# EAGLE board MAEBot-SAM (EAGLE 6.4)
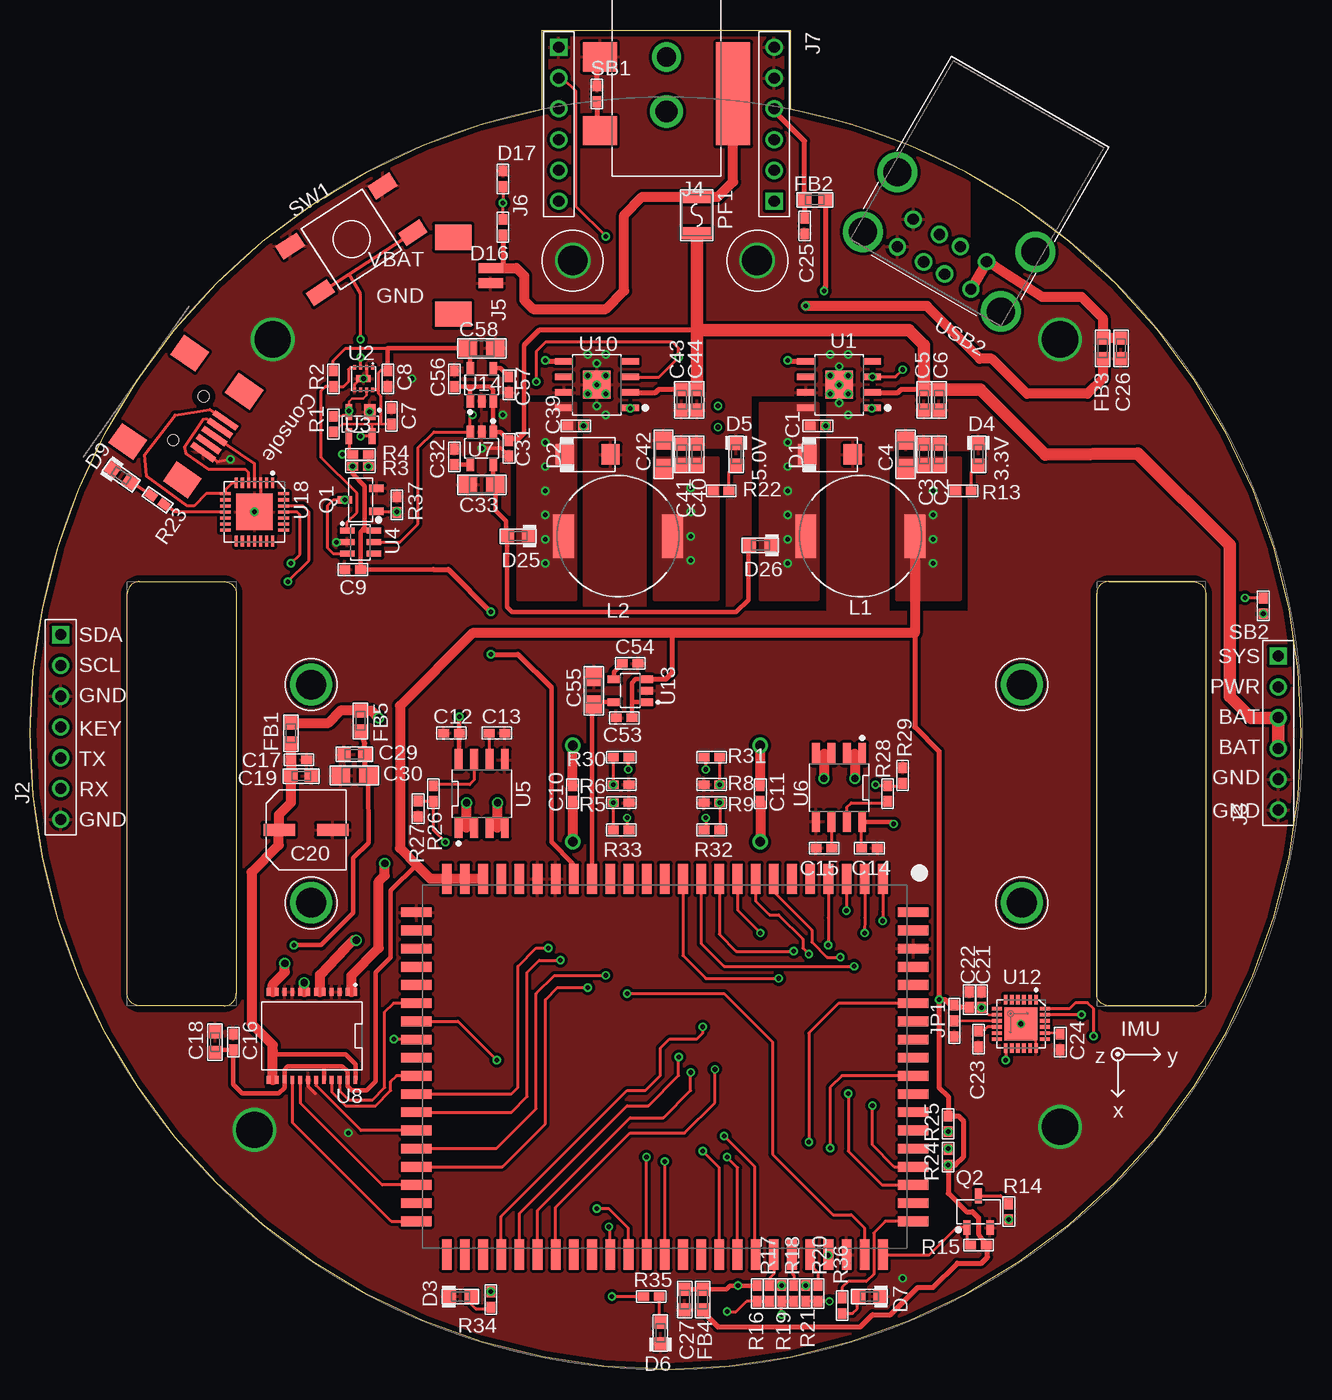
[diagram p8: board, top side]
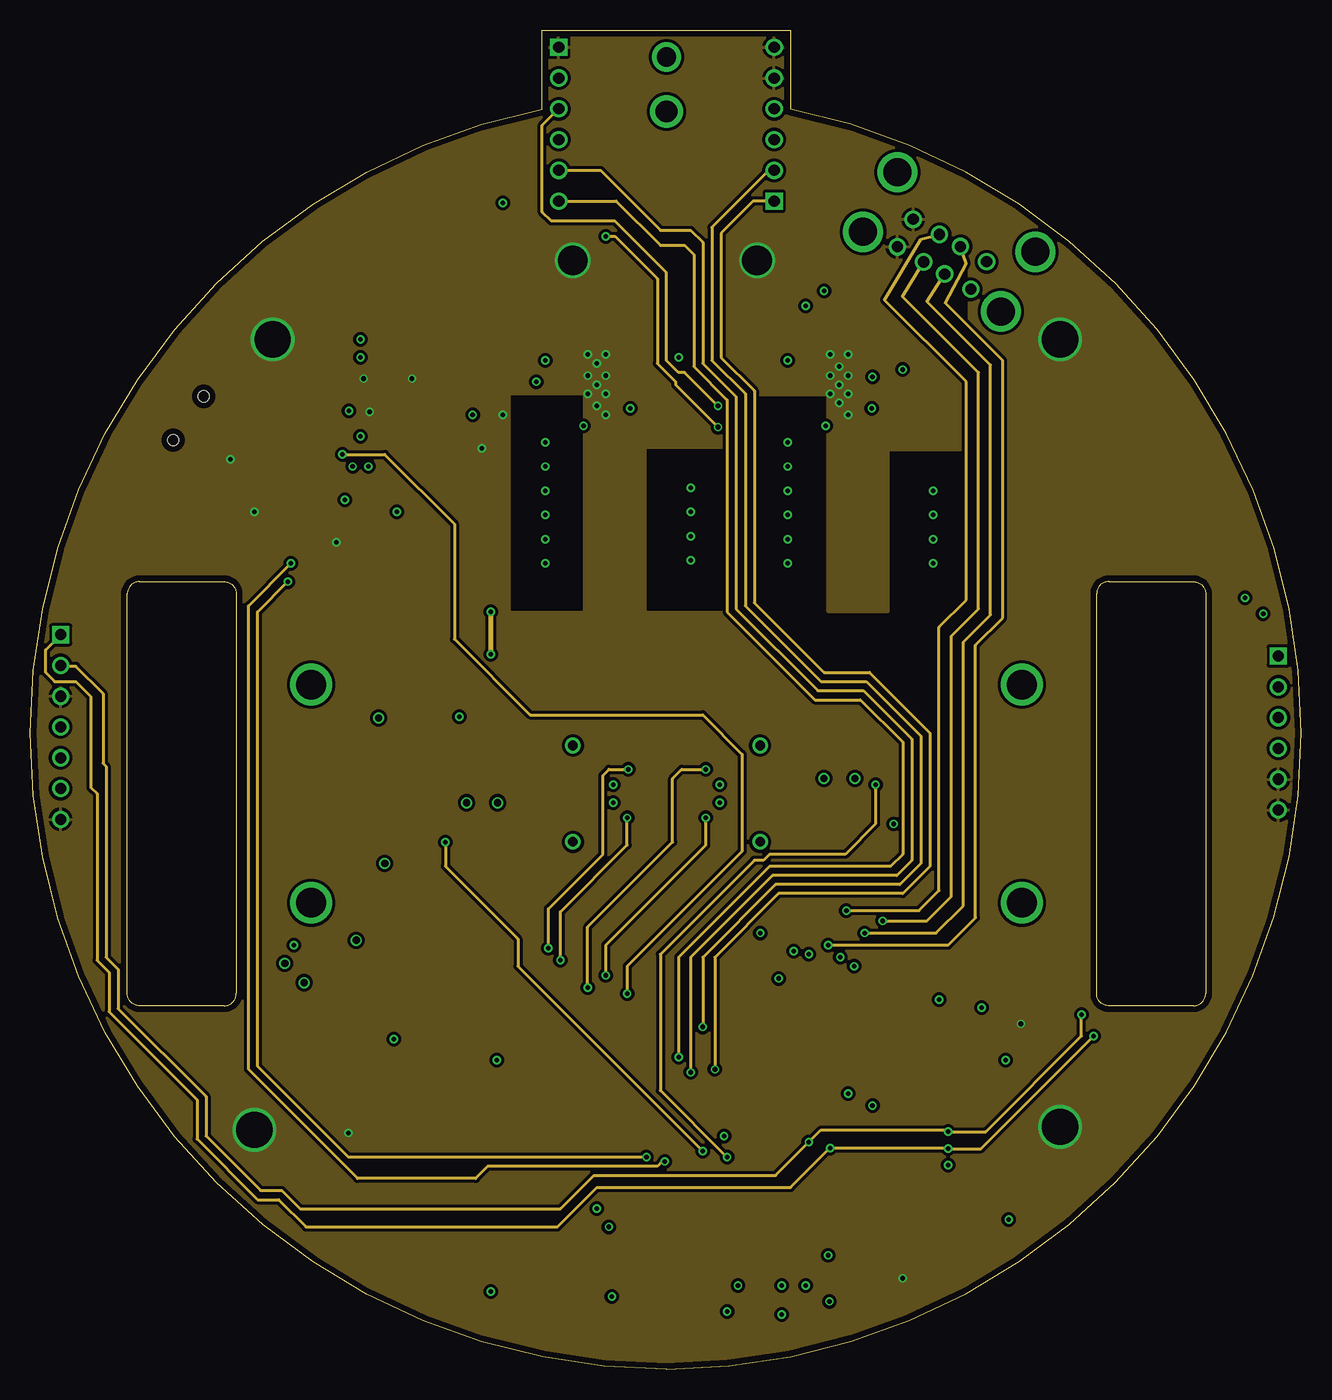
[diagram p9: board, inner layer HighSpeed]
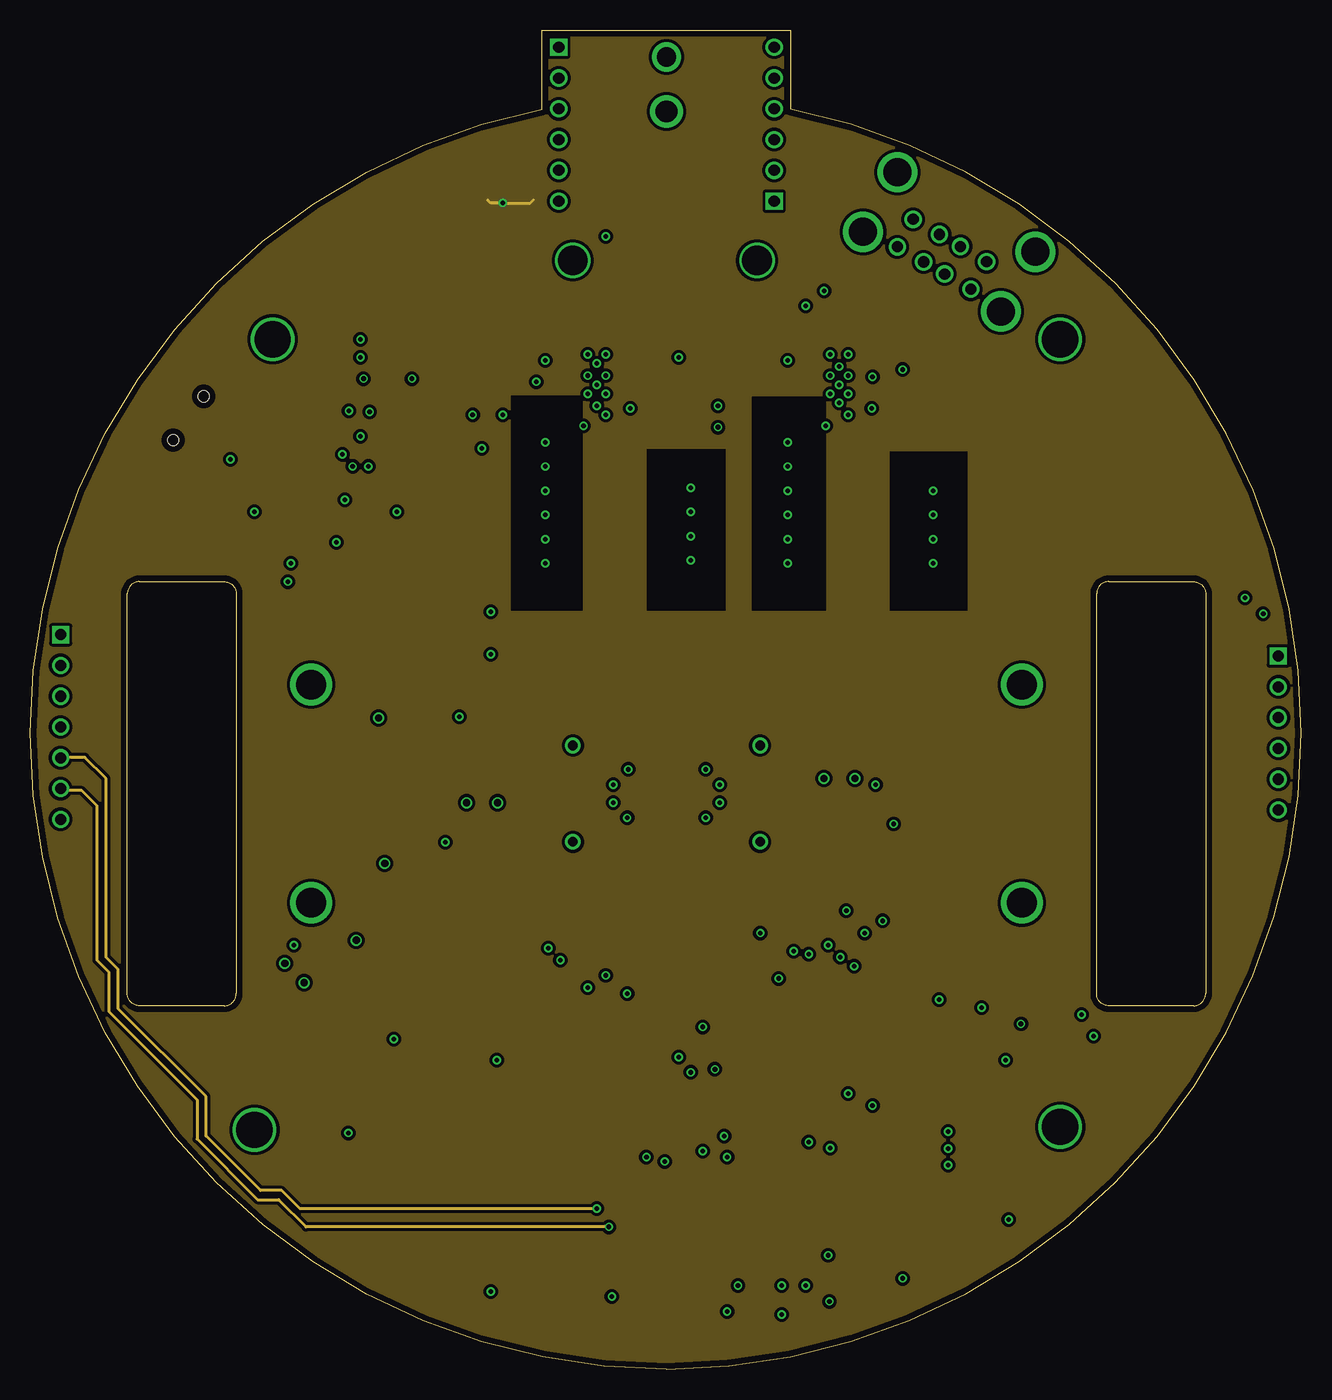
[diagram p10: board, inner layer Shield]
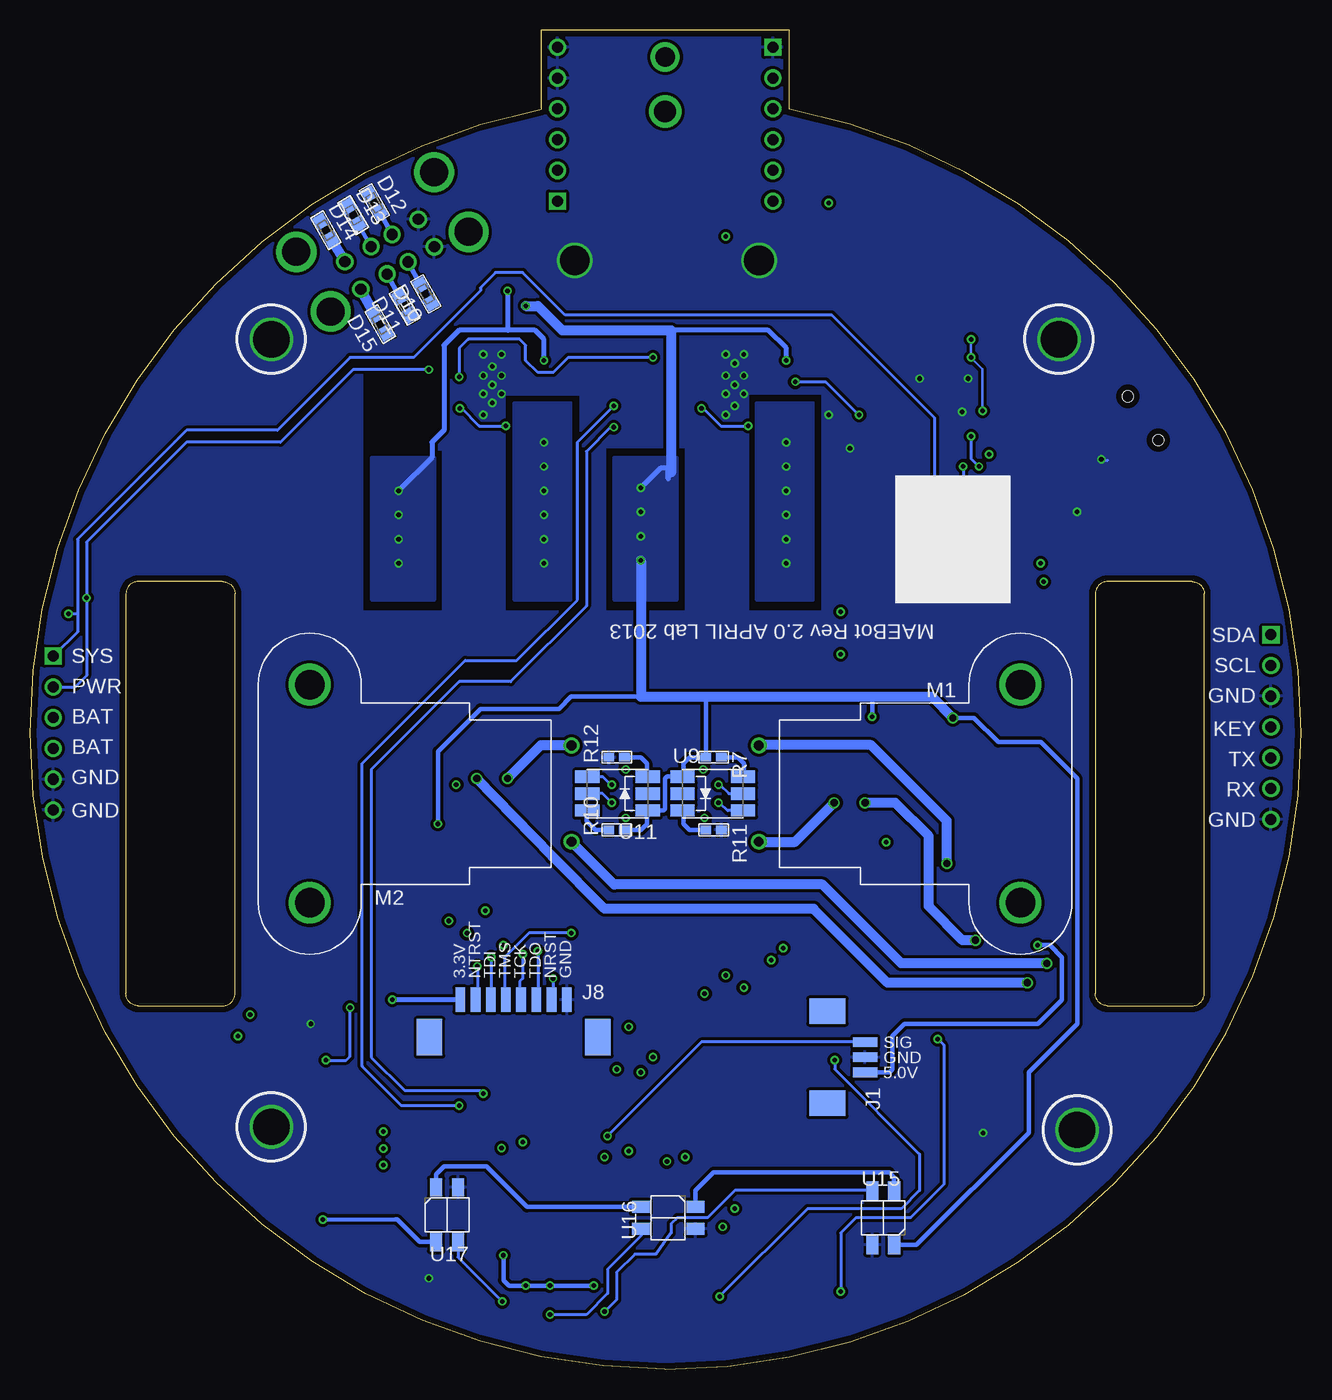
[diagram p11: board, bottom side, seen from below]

Size 104.9 x 110.5 mm. Coordinates in mm from the lower left corner, seen from the top.
Outline: 9.01,65 16.01,65 arc-90 17.01,64 17.01,31 arc-90 16.01,30 9.01,30 arc-90 8.01,31 8.01,64 arc-90 9.01,65
Outline: 89.01,65 96.01,65 arc-90 97.01,64 97.01,31 arc-90 96.01,30 89.01,30 arc-90 88.01,31 88.01,64 arc-90 89.01,65
Outline: 42.26,104 42.26,110.5 62.76,110.5 62.76,104 arc-168 52.51,0 arc-169 42.26,104
Copper layers (1*2+15*16): Top 0.035mm / dielectric 0.15mm / HighSpeed 0.035mm / dielectric 1.1mm / Shield 0.035mm / dielectric 0.15mm / Bottom 0.035mm
Design rules "default *": minimum track width 6mil, minimum drill 15mil, track to track 6mil, track to pad 6mil, pad to pad 6mil, via to via 6mil, smd to smd 0mil, copper to edge 20mil, drill to drill 8mil, minimum pad ring 10mil, minimum via ring 6mil, stop-mask expansion 0mil, vias tented up to drill 16mil, thermal gap 10mil

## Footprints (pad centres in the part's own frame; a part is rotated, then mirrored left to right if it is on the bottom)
R0402 = smd 0.711 x 0.889: P$1 0,0.648; P$2 0,-0.648
SM0603 = smd 1.1 x 1: P$1 -0.85,0; P$2 0.85,0
SM0805 = smd 1.4 x 1.52: P$1 0,1.14; P$2 0,-1.14
VS_SERIES_D8 = smd 2.6 x 1: N 2.2,0; P -2.2,0
SSA33L = smd 1.52 x 1.68: AN -1.88,0; CATH 1.88,0
D0603 = smd 1 x 1.09: AN 0,-0.89; CATH 0,0.89
PICO-3 = smd 2.1 x 3: M$1 -3.8,-3.1; M$2 3.8,-3.1 | smd 0.8 x 2: P$1 -1.25,0; P$2 0,0; P$3 1.25,0
J7X1 = drill 0.914 square: P$1 0,7.62 | drill 0.914: P$2 0,5.08; P$3 0,2.54; P$4 0,0; P$5 0,-2.54; P$6 0,-5.08; P$7 0,-7.62
J6X1 = drill 0.914 square: P$1 0,6.35 | drill 0.914: P$2 0,3.81; P$3 0,1.27; P$4 0,-1.27; P$5 0,-3.81; P$6 0,-6.35
PJ-002A-SMT = drill 1.6: M$1 0,-3.05 | drill 1.8: M$2 0,1.45 | smd 2.8 x 8.5: P$1 -5.5,0 | smd 2.8 x 2.4: P$2 5.5,-3.05; P$3 5.5,3.05
PICO-2 = smd 2.1 x 3: M$1 -3.175,-3.1; M$2 3.175,-3.1 | smd 0.8 x 2: P$1 -0.625,0; P$2 0.625,0
PICO-8 = smd 2.1 x 3: M$1 -6.945,-3.1; M$2 6.945,-3.1 | smd 0.8 x 2: P$1 -4.395,0; P$2 -3.145,0; P$3 -1.895,0; P$4 -0.645,0; P$5 0.605,0; P$6 1.855,0; P$7 3.125,0; P$8 4.395,0
JP0402 = smd 0.711 x 0.889: IN 0,0; OUT1 0,1.296; OUT2 0,-1.296
VLF10040_SERIES = smd 1.7 x 3.6: P$1 -4.5,0; P$2 4.5,0
MMG_MOTOR = drill 0.8: P$1 -3.97,0; P$2 3.97,0 | drill 2.44: P$3 9,-21.6; P$4 -9,-21.6
1210L_SERIES = smd 1 x 2.5: P$1 -1.5,0; P$2 1.5,0
SOT23 = smd 0.6 x 1.2: P$1 -0.95,-1.31; P$2 0.95,-1.31; P$3 0,1.31
SAMA5_CARRIER = smd 0.8 x 2.5: P$1 2,-0.5; P$2 3.5,-0.5; P$3 5,-0.5; P$4 6.5,-0.5; P$5 8,-0.5; P$6 9.5,-0.5; P$7 11,-0.5; P$8 12.5,-0.5; P$9 14,-0.5; P$10 15.5,-0.5; P$11 17,-0.5; P$12 18.5,-0.5; P$13 20,-0.5; P$14 21.5,-0.5; P$15 23,-0.5; P$16 24.5,-0.5; P$17 26,-0.5; P$18 27.5,-0.5; P$19 29,-0.5; P$20 30.5,-0.5; P$21 32,-0.5; P$22 33.5,-0.5; P$23 35,-0.5; P$24 36.5,-0.5; P$25 38,-0.5; P$44 38,30.5; P$45 36.5,30.5; P$46 35,30.5; P$47 33.5,30.5; P$48 32,30.5; P$49 30.5,30.5; P$50 29,30.5; P$51 27.5,30.5; P$52 26,30.5; P$53 24.5,30.5; P$54 23,30.5; P$55 21.5,30.5; P$56 20,30.5; P$57 18.5,30.5; P$58 17,30.5; P$59 15.5,30.5; P$60 14,30.5; P$61 12.5,30.5; P$62 11,30.5; P$63 9.5,30.5; P$64 8,30.5; P$65 6.5,30.5; P$66 5,30.5; P$67 3.5,30.5; P$68 2,30.5 | smd 2.5 x 0.8: P$26 40.5,2.25; P$27 40.5,3.75; P$28 40.5,5.25; P$29 40.5,6.75; P$30 40.5,8.25; P$31 40.5,9.75; P$32 40.5,11.25; P$33 40.5,12.75; P$34 40.5,14.25; P$35 40.5,15.75; P$36 40.5,17.25; P$37 40.5,18.75; P$38 40.5,20.25; P$39 40.5,24.75; P$40 40.5,23.25; P$41 40.5,21.75; P$42 40.5,26.25; P$43 40.5,27.75; P$69 -0.5,27.75; P$70 -0.5,26.25; P$71 -0.5,24.75; P$72 -0.5,23.25; P$73 -0.5,21.75; P$74 -0.5,20.25; P$75 -0.5,18.75; P$76 -0.5,17.25; P$77 -0.5,15.75; P$78 -0.5,14.25; P$79 -0.5,12.75; P$80 -0.5,11.25; P$81 -0.5,9.75; P$82 -0.5,8.25; P$83 -0.5,6.75; P$84 -0.5,5.25; P$85 -0.5,3.75; P$86 -0.5,2.25
FSMJSMA = smd 1.3 x 2.1: P$1 -2.3,4.55; P$2 -2.3,-4.55; P$3 2.3,4.55; P$4 2.3,-4.55
RD-8-1 = smd 0.55 x 1.49: P$1 -1.92,-2.72; P$2 -0.64,-2.72; P$3 0.64,-2.72; P$4 1.92,-2.72; P$5 1.92,2.72; P$6 0.64,2.72; P$7 -0.64,2.72; P$8 -1.92,2.72 | smd 2.29 x 2.29: P$9 0,0
MLF8 = smd 0.35 x 0.25: P$1 -0.925,0.75; P$2 -0.925,0.25; P$3 -0.925,-0.25; P$4 -0.925,-0.75; P$5 0.925,-0.75; P$6 0.925,-0.25; P$7 0.925,0.25; P$8 0.925,0.75 | smd 0.6 x 1.2: P$9 0,0
90-0183 = smd 0.94 x 1.31: P$1 -0.765,-1 | smd 0.55 x 1.31: P$2 0.96,-1; P$3 0.96,1; P$4 -0.96,1
90-0240 = smd 1.2 x 0.5: P$1 -1.1,0.95; P$2 -1.1,0; P$3 -1.1,-0.95; P$4 1.1,-0.95; P$5 1.1,0; P$6 1.1,0.95
LC_8-PIN_SOIC = smd 0.65 x 1.75: P$1 -1.905,-2.8; P$2 -0.635,-2.8; P$3 0.635,-2.8; P$4 1.905,-2.8; P$5 1.905,2.8; P$6 0.635,2.8; P$7 -0.635,2.8; P$8 -1.905,2.8
R-PDS0-G5_(SOT23-5) = smd 0.6 x 1.05: P$1 -0.95,-1.35; P$2 0,-1.35; P$3 0.95,-1.35; P$4 0.95,1.35; P$5 -0.95,1.35
SSOP24-P-300-0.65A = smd 0.32 x 0.65: P$1 -3.575,-3.625; P$2 -2.925,-3.625; P$3 -2.275,-3.625; P$4 -1.625,-3.625; P$5 -0.975,-3.625; P$6 -0.325,-3.625; P$7 0.325,-3.625; P$8 0.975,-3.625; P$9 1.625,-3.625; P$10 2.275,-3.625; P$11 2.925,-3.625; P$12 3.575,-3.625; P$13 3.575,3.625; P$14 2.925,3.625; P$15 2.275,3.575; P$16 1.625,3.625; P$17 0.975,3.625; P$18 0.325,3.625; P$19 -0.325,3.625; P$20 -0.975,3.625; P$21 -1.625,3.625; P$22 -2.275,3.625; P$23 -2.925,3.625; P$24 -3.575,3.625
EE-SX1131 = smd 2 x 1: AN -2.5,1.4; C 2.5,1.4; CA -2.5,-1.4; E1 2.5,0; E2 2.5,-1.4; NC -2.5,0
MPU-60X0 = smd 0.8 x 0.3: P$1 -2,1.25; P$2 -2,0.75; P$3 -2,0.25; P$4 -2,-0.25; P$5 -2,-0.75; P$6 -2,-1.25; P$13 2,-1.25; P$14 2,-0.75; P$15 2,-0.25; P$16 2,0.25; P$17 2,0.75; P$18 2,1.25 | smd 0.3 x 0.8: P$7 -1.25,-1.975; P$8 -0.75,-1.975; P$9 -0.25,-1.975; P$10 0.25,-1.975; P$11 0.75,-1.975; P$12 1.25,-1.975; P$19 1.25,1.975; P$20 0.75,1.975; P$21 0.25,1.975; P$22 -0.25,1.975; P$23 -0.75,1.975; P$24 -1.25,1.975 | smd 2.7 x 2.7: P$25 0,0
ADP171X_(SOT23-5) = smd 0.6 x 1.05: P$1 -0.95,-1.35; P$2 0,-1.35; P$3 0.95,-1.35; P$4 0.95,1.35; P$5 -0.95,1.35
QRE1113GR = smd 1 x 1.5: P$1 0.9,-2.25; P$2 0.9,2.25; P$3 -0.9,2.25; P$4 -0.9,-2.25
28QFN-5MM = smd 0.9 x 0.25: P$1 -2.4,1.5; P$2 -2.4,1; P$3 -2.4,0.5; P$4 -2.4,0; P$5 -2.4,-0.5; P$6 -2.4,-1; P$7 -2.4,-1.5; P$15 2.4,-1.5; P$16 2.4,-1; P$17 2.4,-0.5; P$18 2.4,0; P$19 2.4,0.5; P$20 2.4,1; P$21 2.4,1.5 | smd 0.25 x 0.9: P$8 -1.5,-2.4; P$9 -1,-2.4; P$10 -0.5,-2.4; P$11 0,-2.4; P$12 0.5,-2.4; P$13 1,-2.4; P$14 1.5,-2.4; P$22 1.5,2.4; P$23 1,2.4; P$24 0.5,2.4; P$25 0,2.4; P$26 -0.5,2.4; P$27 -1,2.4; P$28 -1.5,2.4 | smd 3 x 3: P$29 0,0
USB_MINI_A = smd 2.3 x 0.5: D_N 7.85,0.8; D_P 7.85,0; GND 7.85,-1.6; ID 7.85,-0.8; VBUS 7.85,1.6 | smd 2.5 x 2: M1 2.25,4.45; M2 7.75,4.45; M3 7.75,-4.45; M4 2.25,-4.45 | hole 0.9: 5.25,2.2; 5.25,-2.2
XM7A-0442-A = drill 0.92: BOT_D_N -1,2.71; BOT_D_P 1,2.71; BOT_GND 3.5,2.71; BOT_VBUS -3.5,2.71; TOP_D_N -1,5.33; TOP_D_P 1,5.33; TOP_GND 3.5,5.33; TOP_VBUS -3.5,5.33 | drill 2.3: M1 -6.57,0; M2 -6.57,5.68; M3 6.57,5.68; M4 6.57,0

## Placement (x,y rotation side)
C1  0.1uF  [R0402]  65.01,77.85 270 top
C2  22uF  [SM0603]  75.01,75.5 270 top
C3  22uF  [SM0603]  73.76,75.5 270 top
C4  47uF  [SM0805]  72.26,75.5 0 top
C5  10uF  [SM0603]  73.76,80 90 top
C6  10uF  [SM0603]  75.01,80 90 top
C7  0.1uF  [R0402]  29.81,78.65 0 top
C8  0.1uF  [R0402]  29.51,81.75 0 top
C9  0.1uF  [R0402]  26.61,66 90 top
C10  0.1uF  [R0402]  44.76,47.5 0 top
C11  0.1uF  [R0402]  60.26,47.5 0 top
C12  0.1uF  [R0402]  34.76,52.5 90 top
C13  1000pF  [R0402]  38.51,52.5 270 top
C14  0.1uF  [R0402]  69.26,43 270 top
C15  1000pF  [R0402]  65.51,43 90 top
C16  0.1uF  [R0402]  16.76,27 0 top
C17  0.1uF  [R0402]  22.16,50.3 270 top
C18  10uF  [SM0603]  15.26,27 270 top
C19  10uF  [SM0603]  22.36,48.95 180 top
C20  220uF  [VS_SERIES_D8]  22.76,44.5 0 top
C21  0.1uF  [R0402]  78.51,30.5 0 top
C22  0.01uF  [R0402]  77.51,30.5 0 top
C23  0.1uF  [R0402]  78.26,27.25 180 top
C24  2200pF  [R0402]  85.01,27 180 top
C25  0.1uF  [R0402]  63.91,94.35 180 top
C26  22uF  [SM0603]  90.01,84.25 90 top
C27  22uF  [SM0603]  54.01,5.75 90 top
C29  10uF  [SM0603]  26.76,50.75 0 top
C30  47uF  [SM0805]  26.76,49 90 top
C31  1uF  [R0402]  39.51,76 180 top
C32  0.01uF  [R0402]  35.01,75.3 0 top
C33  10uF  [SM0805]  37.26,73 90 top
C39  0.1uF  [R0402]  45.01,77.85 270 top
C40  22uF  [SM0603]  55.01,75.5 270 top
C41  22uF  [SM0603]  53.76,75.5 270 top
C42  47uF  [SM0805]  52.26,75.5 0 top
C43  10uF  [SM0603]  53.76,80 90 top
C44  10uF  [SM0603]  55.01,80 90 top
C53  2.2uF, 6.3V, X5R  [R0402]  49.01,53.75 90 top
C54  0.01uF  [R0402]  49.51,58.25 270 top
C55  2.2uF, 6.3V, X5R  [SM0805]  46.51,56 0 top
C56  1uF  [R0402]  35.01,81.75 0 top
C57  0.01uF  [R0402]  39.51,81.25 180 top
C58  10uF  [SM0805]  37.26,84.25 270 top
D1  SSA33L  [SSA33L]  66.01,75.5 180 top
D2  SSA33L  [SSA33L]  46.01,75.5 180 top
D3  GRN  [D0603]  35.51,6 90 top
D4  GRN  [D0603]  78.26,75.5 0 top
D5  GRN  [D0603]  58.26,75.5 0 top
D6  GRN  [D0603]  52.01,3 180 top
D7  GRN  [D0603]  69.26,6 270 top
D9  BLUE  [D0603]  7.51,73.75 55 top
D10  PGB1010603MR  [SM0603]  72.26,88.75 120 bottom
D11  PGB1010603MR  [SM0603]  74.01,87.75 120 bottom
D12  PGB1010603MR  [SM0603]  76.51,96.25 300 bottom
D13  PGB1010603MR  [SM0603]  78.26,95.25 300 bottom
D14  PGB1010603MR  [SM0603]  80.51,94 300 bottom
D15  PGB1010603MR  [SM0603]  76.01,86.25 120 bottom
D16  PGB1010402KR  [R0402]  39.01,94.25 180 top
D17  PGB1010402KR  [R0402]  39.01,98.25 0 top
D25  [D0603]  40.26,68.75 270 top
D26  [D0603]  60.26,68 270 top
FB1  200R 2.2A  [SM0603]  21.51,52.5 90 top
FB2  200R 2.2A  [SM0603]  64.76,96.5 180 top
FB3  200R 2.2A  [SM0603]  88.51,84.25 90 top
FB4  200R 2.2A  [SM0603]  55.51,5.75 90 top
FB5  200R 2.2A  [SM0603]  27.26,53.5 270 top
J1  IR Range Finder  [PICO-3]  36.01,25.75 270 bottom
J2  To Variscite  [J7X1]  2.51,53 0 top
J3  POWER  [J6X1]  103.01,52.5 0 top
J4  PJ-002A-SMT  [PJ-002A-SMT]  52.51,105.25 180 top
J5  Battery IN  [PICO-2]  38.01,90.25 270 top
J6  Radio-A  [J6X1]  43.62,102.75 0 top
J7  Radio-B  [J6X1]  61.4,102.75 180 top
J8  JTAG  [PICO-8]  65.01,30.5 0 bottom
JP1  JP0402  [JP0402]  76.26,28.75 180 top
L1  3.3uH  [VLF10040_SERIES]  68.51,68.75 0 top
L2  3.3uH  [VLF10040_SERIES]  48.51,68.75 0 top
M1  50:1  [MMG_MOTOR]  44.78,47.5 270 top
M2  50:1  [MMG_MOTOR]  60.24,47.5 90 top
PF1  1210L200 - 4A  [1210L_SERIES]  55.01,95.25 270 top
Q1  2N7002  [SOT23]  27.26,71.75 90 top
Q2  2N7002  [SOT23]  78.26,13 0 top
R1  20K  [R0402]  25.01,78 0 top
R2  10K  [R0402]  25.01,81.75 180 top
R3  100K  [R0402]  27.26,74.5 270 top
R4  10K  [R0402]  27.26,75.5 270 top
R5  6.8K  [R0402]  48.76,46.75 270 top
R6  6.8K  [R0402]  48.76,48.25 270 top
R7  0  [R0402]  48.51,50.5 270 bottom
R8  6.8K  [R0402]  56.26,48.25 90 top
R9  6.8K  [R0402]  56.26,46.75 90 top
R10  0  [R0402]  56.51,44.5 90 bottom
R11  384  [R0402]  48.51,44.5 270 bottom
R12  384  [R0402]  56.51,50.5 90 bottom
R13  56  [R0402]  77.01,72.5 270 top
R14  220  [R0402]  80.76,13 0 top
R15  100K  [R0402]  78.26,10.25 90 top
R16  47K  [R0402]  60.01,6.25 180 top
R17  0  [R0402]  61.01,6.25 180 top
R18  0  [R0402]  63.01,6.25 180 top
R19  47K  [R0402]  62.01,6.25 180 top
R20  0  [R0402]  65.01,6.25 180 top
R21  47K  [R0402]  64.01,6.25 180 top
R22  56  [R0402]  57.01,72.5 270 top
R23  82  [R0402]  10.51,71.75 235 top
R24  4.7K  [R0402]  75.76,17.5 0 top
R25  4.7K  [R0402]  75.76,20.25 180 top
R26  TBD  [R0402]  33.26,47.5 0 top
R27  TBD  [R0402]  32.01,46.25 180 top
R28  TBD  [R0402]  70.76,47.5 0 top
R29  TBD  [R0402]  72.01,49 180 top
R30  0  [R0402]  48.76,50.5 90 top
R31  0  [R0402]  56.26,50.5 270 top
R32  0  [R0402]  56.26,44.5 270 top
R33  0  [R0402]  48.76,44.5 90 top
R34  56  [R0402]  38.01,5.75 180 top
R35  56  [R0402]  51.26,6 270 top
R36  56  [R0402]  67.01,5.25 180 top
R37  100K  [R0402]  30.26,71.35 0 top
SAMA1  SAMA5_CARRIER  [SAMA5_CARRIER]  72.37,39.96 180 top
SB1  SB0402  [R0402]  46.76,105.25 0 top
SB2  SB0402  [R0402]  101.76,63 180 top
SW1  FSMSMTR  [FSMJSMA]  26.51,93.25 303 top
U1  ADP2303ADRZ-3.3-R7  [RD-8-1]  66.76,81.25 90 top
U2  MIC2788  [MLF8]  27.51,81.75 270 top
U3  MAX6816  [90-0183]  27.26,78 180 top
U4  MAX16045  [90-0240]  27.26,68.25 0 top
U5  ACS714 +/- 5A  [LC_8-PIN_SOIC]  37.26,47.5 0 top
U6  ACS714 +/- 5A  [LC_8-PIN_SOIC]  66.76,48 180 top
U7  LP2985-50DBVR  [R-PDS0-G5_(SOT23-5)]  37.26,76 180 top
U8  TB6612FNG  [SSOP24-P-300-0.65A]  23.26,27.5 180 top
U9  EE-SX1131  [EE-SX1131]  48.58,47.5 0 bottom
U10  ADP2303ADRZ-5.0-R7  [RD-8-1]  46.76,81.25 90 top
U11  EE-SX1131  [EE-SX1131]  56.44,47.5 180 bottom
U12  MPU-6050  [MPU-60X0]  81.76,28.5 270 top
U13  ADP1713AUJZ-2.5-R7  [ADP171X_(SOT23-5)]  49.51,56 90 top
U14  LP2985-33DBVR  [R-PDS0-G5_(SOT23-5)]  37.26,81.25 0 top
U15  QRE1113GR  [QRE1113GR]  34.51,12.5 0 bottom
U16  QRE1113GR  [QRE1113GR]  52.26,12.5 90 bottom
U17  QRE1113GR  [QRE1113GR]  70.51,12.75 180 bottom
U18  CP2102  [28QFN-5MM]  18.51,70.75 270 top
USB1  USB_MINI_A  [USB_MINI_A]  8.76,81.5 325 top
USB2  XM7A-0442-A  [XM7A-0442-A]  77.26,95.5 150 top

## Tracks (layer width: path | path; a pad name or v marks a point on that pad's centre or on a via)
3.3V  (via drill 0.38)
  Top 0.203: U12.P$8 79.11,29.25 C21.P$2
  Top 0.254: C22.P$2 C21.P$2 | U12.P$13 v80.51,25.5
  Top 0.381: C53.P$2 49.65,54.75 | 49.65,54.75 49.65,56.65 49.96,56.95 U13.P$3 | U13.P$1 49.7,55.05 49.65,54.75 | 24.26,25 25.76,25 26.18,24.57 U8.P$23 26.18,23.32 26.51,23 27.76,23 28.51,23.75 28.51,32.75 29.76,34 29.76,39.5 31.88,41.62 | 24.26,25 21.26,25 20.98,24.73 U8.P$15 20.98,23.23 20.51,22.75 17.51,22.75 16.76,23.5 C16.P$2 15.46,26.35 C18.P$2 | U8.P$20 24.23,24.98 24.26,25
  Top 0.406: U1.P$5 62.59,83.17 v62.51,83.25 | FB2.P$1 65.61,89.35 v65.51,89 | R24.P$2 76.36,16.85 77.01,17.5 77.01,20.5 76.61,20.9 R25.P$2 75.76,22.5 75.01,23.25 v75.01,30.5 | U13.P$3 52.46,56.95 53.01,57.5 53.01,60.75 | 73.01,60.75 73.01,53 75.01,51 v75.01,30.5 | C22.P$2 76.45,29.85 JP1.OUT2 75.96,30.05 75.51,30.5 v75.01,30.5 | R24.P$2 75.76,14.5 77.26,13 77.76,13 78.26,12.5 78.26,11.15 R15.P$2 79.01,10.15 79.01,9.25 78.51,8.75 76.51,8.75 74.51,6.75 73.26,6.75 71.01,4.5 69.51,4.5 68.51,3.5 56.76,3.5 55.51,4.75 FB4.P$1 | R24.P$2
  Top 0.813: SAMA1.P$23 SAMA1.P$24 SAMA1.P$25 34.33,40.5 33.01,40.5 31.88,41.62 30.51,43 30.51,54.75 36.51,60.75 53.01,60.75 73.01,60.75 L1.P$2
  Bottom 0.254: v80.51,25.5 78.82,25.5 78.51,25.82 C21.P$2
  Bottom 0.406: v62.51,83.25 62.51,85 63.26,85.75 65.51,85.75 | 65.51,85.75 69.51,85.75 70.76,84.5 70.76,77.5 71.76,76.5 71.76,75.25 v74.51,72.5 | v65.51,89 65.51,85.75 | J8.P$1 v75.01,30.5
  other vias: 74.51,70.5 74.51,68.5 74.51,66.5 78.51,29.85 75.76,16.85
  pour Top (no thermals): 71.51,75.25 76.76,75.25 76.76,63.5 71.51,63.5
  pour Bottom (no thermals): 71.51,75.25 76.76,75.25 76.76,63.5 71.51,63.5
3.3V_BYP
  Top 0.381: U14.P$4 38.8,82.6 C57.P$2
5.0V  (via drill 0.38, 0.6)
  Top 0.254: C14.P$2 68.61,45.15 U6.P$8
  Top 0.381: v35.41,53.85 v35.4,53.85 C12.P$2 35.4,50.35 U5.P$8 | 68.61,45.15 71.11,45.15 v71.26,45
  Top 0.406: U10.P$5 42.59,83.17 v42.51,83.25
  Top 0.813: FB3.P$1 88.51,81.75 87.26,80.5 82.26,80.5 79.36,83.4 78.36,83.4 74.01,87.75 v64.01,87.75 | v28.76,53.75 28.16,54.35 FB5.P$1 25.61,54.35 24.61,53.35 FB1.P$2
  Bottom 0.381: R10.P$2 54.51,44.5 54.01,45 54.01,46.03 U11.AN 52.66,46.1 52.51,46.25 52.51,48.75 52.36,48.9 U9.AN 51.01,48.97 51.01,50 50.51,50.5 R7.P$2 49.15,55.4 49.26,55.5 | v35.41,53.85 35.41,55.4 35.51,55.5 | v71.26,45 71.26,51 67.76,54.5 61.26,54.5 60.26,55.5 54.26,55.5 | v28.76,53.75 27.01,53.75 25.01,51.75 21.51,51.75 18.51,48.75 18.51,28.5 22.51,24.5 22.51,19.5 31.76,10.25 U15.P$1
  Bottom 0.406: v42.51,83.25 42.51,84.25 44.01,85.75 52.01,85.75 | 52.01,74 52.26,73.5 C42.P$2 52.9,74.36 v54.51,72.75
  Bottom 0.813: 52.01,74 52.01,85.75 61.01,85.75 63.01,87.75 v64.01,87.75 | v54.51,66.75 54.51,55.5 54.26,55.5 49.26,55.5 35.51,55.5 30.51,55.5 v28.76,53.75
  other vias: 54.51,70.75 54.51,68.75
  pour Top (no thermals): 51.51,75.25 56.76,75.25 56.76,63.5 51.51,63.5
  pour Bottom (no thermals): 51.51,75.25 56.76,75.25 56.76,63.5 51.51,63.5
5.0V_BYP
  Top 0.381: U7.P$4 35.71,74.65 C32.P$2
ADVREF  (via drill 0.38)
  Top 0.381: R19.P$2 | R21.P$2 | R16.P$2 v58.41,6.9 57.76,6.9 57.46,6.6 FB4.P$2 C27.P$2 | SAMA1.P$65 v65.87,9.39 v65.86,9.4
  Bottom 0.381: v58.41,6.9 R19.P$2 R21.P$2 65.41,6.9 65.86,7.35 v65.86,9.4
  other vias: 62.01,6.9 64.01,6.9
BST  (via drill 0.38)
  Top 0.254: U1.P$1 69.38,79.33 v69.46,79.3 | C1.P$1
  Bottom 0.254: v69.46,79.3 69.36,79.35 67.86,77.85 C1.P$1
  other vias: 65.66,77.85
BST1  (via drill 0.38)
  Top 0.254: U10.P$1 v49.51,79.3 | C39.P$1
  Bottom 0.254: v49.51,79.3 49.41,79.35 47.91,77.85 C39.P$1
  other vias: 45.66,77.85
BTN_LONG_PRESS
  Top 0.254: U2.P$4 26.43,82.67 26.26,82.5 26.26,81.5 25.86,81.1 R2.P$1 24.36,81.1 24.01,80.75 24.01,75.25 26.96,72.3 26.96,70.7 26.16,69.9 U4.P$1
BTN_PRESS  (via drill 0.38)
  Top 0.203: R1.P$1 25.7,78.65 25.81,78.75 26.26,78.75 26.3,78.79 U3.P$2 | U2.P$7 27.76,80.4 27.46,80.1 26.56,80.1 26.31,79.85 v26.31,79.1
  Top 0.254: U3.P$2 v26.31,79.1 | U2.P$3 v27.26,83.5 | SW1.P$4 26.33,90.39 | 26.33,90.39 SW1.P$3 | v27.26,85 27.26,88.75 26.33,90.39
  Bottom 0.203: v27.26,85 v27.26,83.5 26.31,82.55 v26.31,79.1
BTN_SHORT_PRESS  (via drill 0.38)
  Top 0.254: U3.P$3 26.3,75.81 R4.P$2 v25.76,75.5 | v49.26,31 57.26,31 61.26,27 61.26,17.75 66.26,12.75 67.76,12.75 68.87,11.64 SAMA1.P$67
  HighSpeed 0.254: v25.76,75.5 29.26,75.5 35.01,69.75 35.01,60.25 41.26,54 55.51,54 58.76,50.75 58.76,42.75 49.26,33.25 v49.26,31
CHG_GND2
  Top 0.406: SB1.P$2 46.76,102.45 J4.P$3
COM_SHIELD  (via drill 0.38)
  Top 0.254: D16.P$2 v39.01,96.25 D17.P$2
  Shield 0.254: 37.76,96.5 38.01,96.25 v39.01,96.25 41.26,96.25 41.51,96.5
  pour Shield (isolate 0.254): 106.51,-1.5 -1.49,-1.5 -1.49,110.5 39.51,110.5 39.51,62.5 77.51,62.5 77.51,109.5 106.51,109.5
  pour Shield (isolate 0.254): 39.51,111.5 39.51,80.5 45.71,80.5 45.71,62.5 50.76,62.5 50.76,76.1 57.51,76.1 57.51,62.55 59.46,62.55 59.46,80.45 65.81,80.45 65.81,62.55 70.81,62.5 70.81,75.85 77.51,75.9 77.51,111.5
CONSOLE_/SUSP
  Top 0.254: U18.P$11 12.01,70.75 R23.P$1
CONSOLE_DM
  Top 0.254: U18.P$5 18.01,74 17.76,74.25 14.76,74.25 12.86,75.55 12.76,76.15 14.26,78.4 14.51,78.45 USB1.D_N
CONSOLE_DP
  Top 0.254: U18.P$4 18.51,74.75 USB1.D_P
CONSOLE_LED
  Top 0.254: R23.P$2 D9.AN
CONSOLE_RX  (via drill 0.38)
  Top 0.254: SAMA1.P$56 v52.37,17.14 v52.36,17.15 | v21.51,66.5 22.26,67.25 22.26,70.5 22.01,70.75 U18.P$25
  HighSpeed 0.254: v52.36,17.15 52.16,17.15 51.76,16.75 37.76,16.75 36.76,15.75 27.01,15.75 26.01,16.75 18.01,24.75 18.01,63 v21.51,66.5
CONSOLE_TX  (via drill 0.38)
  Top 0.254: SAMA1.P$55 v50.87,17.49 v50.86,17.5 | v21.26,65 23.01,66.75 23.01,70.75 22.51,71.25 U18.P$26
  HighSpeed 0.254: v50.86,17.5 26.26,17.5 18.76,25 18.76,62.5 v21.26,65
CONSOLE_VBUS
  Top 0.254: USB1.VBUS 14.81,79.2 11.96,78.75 9.46,75.5 9.61,73.7 13.01,71.25 13.51,71.25 14.51,72.25 U18.P$8 16.11,72.6 16.66,73.15 U18.P$7
CS_FLTR_1
  Top 0.254: U5.P$6 37.89,52.47 C13.P$2
CS_FLTR_2
  Top 0.254: C15.P$2 66.15,45.17 U6.P$6
GND  (via drill 0.38, 2.44, 3)
  Top 0.203: U12.P$18 83.01,27.25 U12.P$25
  Top 0.254: U2.P$2 27.76,82 U2.P$9 27.26,81.75 26.76,81.25 U2.P$5 | U18.P$3 19.01,71.25 U18.P$29 | USB1.GND 15.41,74.9 v16.51,75.1 | U4.P$2 v25.26,68.25
  Top 0.305: v37.26,76 38.86,76 C31.P$1 | U8.P$18 22.93,23.32 23.51,22.75
  Top 0.406: SB1.P$1 46.76,108.05 J4.P$2
  Bottom 0.254: v16.51,75.1 16.01,75 | v25.26,68.25 25.26,68.75
  other vias: 18.51,70.75 27.51,81.75 28.01,79 46.76,81.25 46.01,82 47.51,82 46.01,80.5 47.51,80.5 46.76,83 46.01,83.75 47.51,83.75 46.76,79.5 47.51,78.75 66.76,81.25 66.01,82 67.51,82 66.01,80.5 67.51,80.5 66.76,82.75 66.01,83.75 67.51,83.75 66.76,79.75 67.51,78.75 81.76,28.5 85.01,20 85.01,85 20.01,85 18.51,19.75 44.76,91.5 59.98,91.5 31.51,81.75 39.01,78.75 26.26,19.5 72.01,7.5
  pour Top (isolate 0.254): 52.51,-1.5 -1.49,-1.5 -1.49,52.5 -1.49,110.5 39.51,110.5 39.51,62.5 77.51,62.5 77.51,109.5 106.51,109.5 106.51,52.5 106.51,-1.5
  pour Bottom (isolate 0.254): 106.51,-1.5 -1.49,-1.5 -1.49,110.5 39.51,110.5 39.51,62.5 77.51,62.5 77.51,109.5 106.51,109.5
  pour HighSpeed (isolate 0.254): 106.51,-1.5 -1.49,-1.5 -1.49,110.5 39.51,110.5 39.51,62.5 77.51,62.5 77.51,109.5 106.51,109.5
  pour Top (isolate 0.254): 39.51,111.5 39.51,80.5 45.71,80.5 45.71,62.5 50.76,62.5 50.76,76.1 57.51,76.1 57.51,62.55 59.46,62.55 59.46,80.45 65.81,80.45 65.81,62.55 70.81,62.5 70.81,75.85 77.51,75.9 77.51,111.5
  pour HighSpeed (isolate 0.254): 39.51,111.5 39.51,80.5 45.71,80.5 45.71,62.5 50.76,62.5 50.76,76.1 57.51,76.1 57.51,62.55 59.46,62.55 59.46,80.45 65.81,80.45 65.81,62.55 70.81,62.5 70.81,75.85 77.51,75.9 77.51,111.5
  pour Bottom (isolate 0.254): 39.51,111.5 39.51,80.5 45.71,80.5 45.71,62.5 50.76,62.45 50.76,76.1 57.51,76.1 57.51,62.5 59.46,62.55 59.46,80.45 65.81,80.45 65.81,62.55 70.81,62.5 70.81,75.85 77.51,75.9 77.51,111.5
I2C_SCL  (via drill 0.38)
  Top 0.254: v86.76,29.25 U12.P$23 | R25.P$1 | SAMA1.P$81 66.72,30.21 64.26,27.75 v64.26,18.75
  HighSpeed 0.254: v86.76,29.25 86.76,27.5 78.86,19.6 R25.P$1 75.61,19.75 65.26,19.75 v64.26,18.75 61.51,16 46.51,16 43.76,13.25 22.26,13.25 20.76,14.75 19.01,14.75 14.51,19.25 14.51,22.5 7.26,29.75 7.26,33 6.26,34 6.26,49.75 6.01,50 6.01,55.75 3.76,58 2.59,58 J2.P$2
  other vias: 75.76,19.6
I2C_SDA  (via drill 0.38)
  Top 0.254: v87.76,27.5 87.76,29.75 87.26,30.25 86.26,30.25 85.76,29.75 U12.P$24 | R24.P$1 v75.76,18.2 | SAMA1.P$77 66.97,24.21 66.01,23.25 v66.01,18.25
  HighSpeed 0.254: v87.76,27.5 78.46,18.2 v75.76,18.2 75.71,18.25 v66.01,18.25 62.76,15 46.76,15 43.51,11.75 22.76,11.75 20.51,14 18.76,14 13.76,19 13.76,22.25 6.51,29.5 6.51,32.75 5.51,33.75 5.51,47.5 5.01,48 5.01,55.5 3.76,56.75 2.01,56.75 1.26,57.5 1.26,59.37 J2.P$1
IND_3.3V
  Top 0.254: R13.P$1 77.66,74 D4.AN
IND_5.0V
  Top 0.254: R22.P$1 57.65,74.01 D5.AN
IRLED_LEFT  (via drill 0.38)
  Top 0.254: R21.P$1 R20.P$1 v65.96,5.6
  Bottom 0.254: U17.P$3 69.61,9.25 v65.96,5.6
IRLED_LEFT_SAM
  Top 0.254: SAMA1.P$64 64.37,8.64 65.01,8 R20.P$2
IRLED_MID  (via drill 0.38)
  Top 0.254: R18.P$1 R19.P$1 v62.01,4.5
  Bottom 0.254: v62.01,4.5 59.01,4.5 57.26,6.25 57.26,8.25 54.51,11 U16.P$3
IRLED_MID_SAM
  Top 0.254: SAMA1.P$63 62.87,7.89 63.01,7.75 R18.P$2
IRLED_ON
  Top 0.254: R15.P$1 77.31,10.55 Q2.P$1 77.25,11.75 76.51,11.75 74.22,9.46 SAMA1.P$68
IRLED_RIGHT  (via drill 0.38)
  Top 0.254: R17.P$1 R16.P$1 59.11,5.6 58.26,4.75 v57.51,4.75
  Bottom 0.254: U15.P$3 46.74,14.77 49.01,12.5 51.51,12.5 52.01,12 52.01,11.25 53.26,9.5 55.01,9.5 56.51,8 56.51,5.75 v57.51,4.75
IRLED_RIGHT_SAM
  Top 0.254: SAMA1.P$62 61.37,7.86 61.01,7.5 R17.P$2
IRLINE_IND_LEFT
  Top 0.254: SAMA1.P$69 70.57,12.21 69.61,11.25 69.61,7.85 69.01,7.25 67.51,7.25 67.01,6.75 R36.P$2
IRLINE_IND_MID  (via drill 0.38)
  Top 0.254: SAMA1.P$32 35.3,28.71 v38.51,25.5 | v48.01,6 R35.P$2
  Bottom 0.254: v38.51,25.5 38.51,24.75 31.51,17.75 31.51,14.75 33.01,13.25 40.76,13.25 v48.01,6
IRLINE_IND_RIGHT  (via drill 0.38)
  Top 0.254: SAMA1.P$33 30.05,27.21 v30.01,27.25 | R34.P$2
  Bottom 0.254: v30.01,27.25 29.51,26.75 29.51,15.25 32.26,12.5 36.76,12.5 38.01,11.25 R34.P$2
  other vias: 38.01,6.4
M1+  (via drill 0.6)
  Top 0.254: U8.P$1 26.51,31.12 U8.P$2
  Top 0.813: 26.51,31.12 26.51,32.5 28.76,34.75 28.76,40.25 29.26,40.75 v29.26,41.75 | C10.P$1 44.76,51.45 M1.P$1
  Bottom 0.813: v29.26,41.75 29.26,45.25 35.51,51.5 44.75,51.5 M1.P$1
M1-  (via drill 0.6)
  Top 0.381: U5.P$4 38.56,44.7 U5.P$3
  Top 0.813: 38.56,44.7 v38.56,46.75 | C10.P$2 44.76,43.55 M1.P$2
  Bottom 0.813: M1.P$2 41.78,43.53 v38.56,46.75
M1-_SENSE  (via drill 0.6)
  Top 0.254: U8.P$6 23.91,31.12 U8.P$5
  Top 0.381: U5.P$2 36.01,44.7 U5.P$1
  Top 0.813: 23.91,31.12 23.91,32.55 26.01,34.75 26.66,35.4 v26.91,35.4 | 36.01,44.7 v36.01,46.75
  Bottom 0.813: v26.91,35.4 27.96,35.4 30.76,38.2 30.76,44 33.51,46.75 v36.01,46.75
M1_CS
  Top 0.254: U5.P$7 36.62,48.62 36.26,48.25 33.36,48.25 R26.P$1
M1_CS_DIV  (via drill 0.38)
  Top 0.254: R27.P$2 32.05,46.85 R26.P$2 33.26,44.5 v34.26,43.5 | v55.51,18 56.87,16.64 SAMA1.P$59
  HighSpeed 0.254: v34.26,43.5 34.26,41.5 40.26,35.5 40.26,33.25 v55.51,18
M1_E1  (via drill 0.38)
  Top 0.254: R30.P$1 R6.P$2
  Bottom 0.254: R6.P$2 48.01,48.25 47.26,47.5 U9.E1
  other vias: 48.11,48.25
M1_E2  (via drill 0.38)
  Top 0.254: R5.P$2 R33.P$1
  Bottom 0.254: R5.P$2 48.01,46.75 47.36,46.1 U9.E2
  other vias: 48.11,46.75
M1_PWM1
  Top 0.254: U8.P$21 24.88,22.88 26.01,21.75 28.51,21.75 29.76,23 29.76,23.75 30.22,24.21 SAMA1.P$35
M1_PWM2
  Top 0.254: U8.P$22 25.53,22.98 26.26,22.25 28.26,22.25 29.26,23.25 29.26,29.5 29.97,30.21 SAMA1.P$31
M1_QUAD_A  (via drill 0.38)
  Top 0.254: SAMA1.P$37 39.72,21.21 41.01,22.5 41.01,32.75 42.01,33.75 v43.76,33.75 | v49.26,45.5 49.26,44.65 R33.P$2
  HighSpeed 0.254: v43.76,33.75 43.76,37.75 49.26,43.25 v49.26,45.5
M1_QUAD_B  (via drill 0.38)
  Top 0.254: SAMA1.P$36 39.72,22.71 40.26,23.25 40.26,33.25 41.76,34.75 v42.76,34.75 | v49.36,49.5 49.36,50.45 R30.P$2
  HighSpeed 0.254: v42.76,34.75 42.76,38 47.26,42.5 47.26,49 47.76,49.5 v49.36,49.5
M2+  (via drill 0.6)
  Top 0.254: U8.P$12 20.01,31.12 U8.P$11
  Top 0.813: 20.01,31.12 20.01,31.75 21.01,32.75 v21.01,33.5 | C11.P$2 60.26,43.55 M2.P$1
  Bottom 0.813: v21.01,33.5 33.01,33.5 39.51,40 56.71,40 M2.P$1
M2-  (via drill 0.6)
  Top 0.381: U6.P$4 65.51,50.8
  Top 0.406: U6.P$3 65.51,50.8
  Top 0.813: 65.51,50.8 v65.51,48.75 | C11.P$1 60.26,51.45 M2.P$2
  Bottom 0.813: v65.51,48.75 62.76,51.5 60.27,51.5 M2.P$2
M2-_SENSE  (via drill 0.6)
  Top 0.254: U8.P$8 22.61,31.12 U8.P$7
  Top 0.381: U6.P$1 68.06,50.8 U6.P$2
  Top 0.813: 22.61,31.12 v22.61,31.9 | 68.06,50.8 v68.06,48.75
  Bottom 0.813: v22.61,31.9 34.16,31.9 40.26,38 57.51,38 61.81,42.3 v68.06,48.75
M2_CS
  Top 0.254: U6.P$7 67.39,46.38 67.76,46.75 70.65,46.75 R28.P$2
M2_CS_DIV  (via drill 0.38)
  Top 0.254: R29.P$1 71.8,48.15 R28.P$1 69.86,48.15 v69.76,48.25 | v57.51,17.5 58.37,16.64 SAMA1.P$60
  HighSpeed 0.254: v69.76,48.25 69.76,45 67.26,42.5 61.01,42.5 60.51,42 59.76,42 52.01,34.25 52.01,23 v57.51,17.5
M2_E1  (via drill 0.38)
  Top 0.254: R9.P$2 R32.P$1
  Bottom 0.254: R9.P$2 57.66,47.5 U11.E1
  other vias: 56.91,46.75
M2_E2  (via drill 0.38)
  Top 0.254: R8.P$2 R31.P$1
  Bottom 0.254: R8.P$2 57.01,48.25 57.66,48.9 U11.E2
  other vias: 56.91,48.25
M2_PWM1
  Top 0.254: U8.P$16 21.63,20.38 29.8,12.21 SAMA1.P$43
M2_PWM2
  Top 0.254: U8.P$17 22.28,21.98 29.05,15.21 SAMA1.P$39
M2_QUAD_A  (via drill 0.38)
  Top 0.254: SAMA1.P$40 38.97,16.71 42.51,20.25 42.51,30.5 43.51,31.5 v46.01,31.5 | v55.76,49.5 55.76,50.35 R31.P$2
  HighSpeed 0.254: v46.01,31.5 46.01,36.5 53.01,43.5 53.01,48.75 53.76,49.5 v55.76,49.5
M2_QUAD_B  (via drill 0.38)
  Top 0.254: v47.51,32.5 43.26,32.5 41.76,31 41.76,21.5 38.47,18.21 SAMA1.P$41 | v55.76,45.5 55.76,44.65 R32.P$2
  HighSpeed 0.254: v47.51,32.5 47.51,35 55.76,43.25 v55.76,45.5
MAIN_PWREN  (via drill 0.38)
  Top 0.254: U4.P$5 30.51,68.25 32.01,69.75 32.01,76.05 33.31,77.35 U7.P$3 36.31,78.55 v36.51,78.75 | U10.P$3 51.9,81.89 v53.51,83.5 53.51,84.25 53.01,84.75 42.51,84.75 41.76,84 v41.76,81.5 | U1.P$3 v69.51,81.9 71.41,81.9 v72.01,82.5 | SB2.P$2 100.96,63.65 v100.26,63.65
  Bottom 0.254: v53.51,83.5 60.51,83.5 61.76,82.25 63.01,82.25 64.01,83.25 64.01,84.5 64.51,85 68.76,85 69.51,84.25 v69.51,81.9 | v41.76,81.5 39.26,81.5 v36.51,78.75 | v72.01,82.5 78.26,82.5 84.26,76.5 92.01,76.5 100.26,68.25 v100.26,63.65 100.26,57.25 101.2,56.31 J3.P$2
MISO  (via drill 0.38)
  Top 0.254: SAMA1.P$50 43.37,13.36 49.51,19.5 54.01,19.5 56.51,22 v56.51,24.75
  HighSpeed 0.254: J7.P$1 59.66,96.4 57.01,93.75 57.01,83.5 59.76,80.75 59.76,63.25 65.51,57.5 69.26,57.5 74.26,52.5 74.26,41.5 72.01,39.25 61.76,39.25 56.51,34 v56.51,24.75
MOSI  (via drill 0.38)
  Top 0.254: SAMA1.P$49 41.87,13.11 49.51,20.75 52.26,20.75 54.51,23 v54.51,24.5
  HighSpeed 0.254: J6.P$5 47.07,98.94 52.01,94 54.51,94 55.51,93 55.51,83 58.26,80.25 58.26,62.75 65.01,56 68.76,56 72.76,52 72.76,42 71.51,40.75 61.26,40.75 54.51,34 v54.51,24.5
MOTOR_STBY
  Top 0.254: U8.P$19 23.58,23.43 27.3,19.71 SAMA1.P$38
MPU_AD
  Top 0.203: U12.P$9 JP1.IN
MPU_CP
  Top 0.203: U12.P$20 84.9,27.75 C24.P$2
MPU_REG
  Top 0.254: U12.P$10 79.01,28.25 78.76,28 78.36,28 C23.P$2
N$1
  Top 0.254: D3.AN 36.4,5.36 36.76,5 37.9,5 R34.P$1
N$2
  Bottom 0.381: R7.P$1 46.51,50.5 46.01,50 46.01,48.97 U9.C
N$3
  Bottom 0.381: R12.P$2 54.51,50.5 54.01,50 54.01,48.97 U11.CA
N$4
  Top 0.254: R35.P$1 51.9,3.99 D6.AN
N$5
  Top 0.254: R36.P$1 67.86,4.6 68.26,5 68.26,5.89 D7.AN
N$6
  Bottom 0.381: U15.P$2 33.61,15.85 34.01,16.25 48.51,16.25 50.01,14.75 U16.P$1
N$7
  Bottom 0.381: R11.P$2 50.51,44.5 51.01,45 51.01,46.03 U9.CA
N$8
  Bottom 0.381: U16.P$2 63.91,13.4 67.26,16.75 70.76,16.75 71.41,16.1 U17.P$1
N$9
  Top 0.254: Q2.P$3 80.09,14.31 R14.P$1
N$10
  Bottom 0.381: R10.P$1 58.26,44.5 59.01,45.25 59.01,46.03 U11.C
N$13  (via drill 0.38)
  Top 0.254: R14.P$2
  Bottom 0.254: 74.74,12.37 74.63,12.37
  Bottom 0.381: 74.74,12.37 R14.P$2 | 74.63,12.37 72.76,10.5 U17.P$2
  other vias: 80.76,12.35
N$66
  Top 0.381: U13.P$4 48.16,57.55 C54.P$2
NRST  (via drill 0.38)
  Top 0.254: SAMA1.P$12 53.87,34.14 55.76,32.25 v61.76,32.25
  Bottom 0.254: v61.76,32.25 61.76,30.62 J8.P$7
NTRST  (via drill 0.38)
  Top 0.254: SAMA1.P$11 55.37,35.14 57.26,33.25 v68.01,33.25
  Bottom 0.254: v68.01,33.25 68.01,30.64 J8.P$2
RAD/CS  (via drill 0.38)
  Top 0.254: SAMA1.P$47 38.87,12.61 49.26,23 50.76,23 52.01,24.25 52.01,26.5 52.76,27.25 55.01,27.25 55.51,27.75 v55.51,28.25
  HighSpeed 0.254: J7.P$2 60.95,98.94 56.26,94.25 56.26,83.25 59.01,80.5 59.01,63 65.26,56.75 69.01,56.75 73.51,52.25 73.51,41.75 71.76,40 61.51,40 55.51,34 v55.51,28.25
RAD_/RST  (via drill 0.38)
  Top 0.254: J6.P$2 43.95,106.56 45.01,105.5 45.01,96 v47.51,93.5 | v67.51,22.75 67.51,18 70.3,15.21 SAMA1.P$71
  HighSpeed 0.254: v47.51,93.5 48.26,93.5 51.76,90 51.76,83 53.26,81.5 53.26,81.25 v56.76,77.75
  Bottom 0.254: v56.76,77.75 57.01,77.75 59.01,75.75 59.01,63 65.26,56.75 69.51,56.75 76.76,49.5 76.76,25.75 74.01,23 67.76,23 v67.51,22.75
RAD_VIN
  Top 0.406: C25.P$2 FB2.P$2 63.91,101.35 61.4,103.86 J7.P$4
RAD_WAKE  (via drill 0.38)
  Top 0.254: v69.51,21.75 69.51,18.5 71.3,16.71 SAMA1.P$72
  HighSpeed 0.254: v56.76,79.5 54.01,82.25 53.51,82.25 52.51,83.25 52.51,90.5 48.26,94.75 43.01,94.75 42.26,95.5 42.26,102.66 J6.P$3
  Bottom 0.254: v69.51,21.75 74.26,21.75 77.51,25 77.51,50 69.01,58.5 64.76,58.5 59.76,63.5 59.76,76.5 v56.76,79.5
SHARP_VOUT  (via drill 0.38)
  Top 0.254: v57.26,19.25 59.76,16.75 59.76,9.57 SAMA1.P$61
  Bottom 0.254: J1.P$1 49.51,27 v57.26,19.25
SOFTPWR_CLR  (via drill 0.38)
  Top 0.254: U4.P$3 25.01,67.3 24.51,67.8 24.51,71.25 25.01,71.75 Q1.P$3 25.95,71.79 v25.96,71.75 | R3.P$1 27.9,74.35 R3.P$1 R4.P$1
  Bottom 0.254: v25.96,71.75 26.71,72.45 27.91,73.65 R3.P$1
  other vias: 27.91,74.5
SPICLK  (via drill 0.38)
  Top 0.254: SAMA1.P$48 40.37,12.86 49.26,21.75 51.01,21.75 53.51,24.25 v53.51,25.75
  HighSpeed 0.254: J6.P$6 48.36,96.4 52.01,92.75 54.01,92.75 54.76,92 54.76,82.75 57.51,80 57.51,62.5 64.76,55.25 68.51,55.25 72.01,51.75 72.01,42.5 71.01,41.5 61.01,41.5 53.51,34 v53.51,25.75
SW_3.3V  (via drill 0.38)
  other vias: 62.51,76.5 62.51,74.5 62.51,72.5 62.51,70.5 62.51,68.5 62.51,66.5
  pour Top (no thermals): 65.01,79.75 65.01,63.5 60.26,63.5 60.26,79.75
  pour Bottom (no thermals): 65.01,79.75 65.01,63.5 60.26,63.5 60.26,79.75
SW_5V  (via drill 0.38)
  other vias: 42.51,76.5 42.51,74.5 42.51,72.5 42.51,70.5 42.51,68.5 42.51,66.5
  pour Top (no thermals): 45.01,79.75 45.01,63.5 40.26,63.5 40.26,79.75
  pour Bottom (no thermals): 45.01,79.75 45.01,63.5 40.26,63.5 40.26,79.75
SYSEN  (via drill 0.38)
  Top 0.254: Q1.P$1 30.21,70.8 v30.26,70.75 R37.P$2 | SB2.P$1 101.8,62.35 SB2.P$1
  Bottom 0.254: v30.26,70.75 30.26,78.5 38.76,87 60.76,87 64.26,90.5 66.51,90.5 67.76,89.25 67.76,89 73.26,83.5 78.51,83.5 84.51,77.5 92.01,77.5 101.01,68.5 101.01,62.35 | 101.01,62.35 101.01,60.85 J3.P$1 | SB2.P$1 101.01,62.35
  other vias: 101.76,62.35
TCK  (via drill 0.38)
  Top 0.254: SAMA1.P$8 59.87,38.64 61.01,37.5 61.76,37.5 63.76,35.5 63.76,34.75 v64.26,34.25
  Bottom 0.254: v64.26,34.25 64.26,32.25 64.51,32 64.51,30.61 J8.P$5
TDI  (via drill 0.38)
  Top 0.254: SAMA1.P$7 61.37,39.39 64.51,36.25 64.51,35.25 65.76,34 v66.86,34
  Bottom 0.254: v66.86,34 66.86,30.55 J8.P$3
TDO  (via drill 0.38)
  Top 0.254: SAMA1.P$10 56.87,35.89 58.26,34.5 v63.01,34.5
  Bottom 0.254: v63.01,34.5 63.01,30.64 J8.P$6
TMS  (via drill 0.38)
  Top 0.254: SAMA1.P$9 58.37,37.89 v60.26,36
  Bottom 0.254: v60.26,36 63.76,36 65.76,34 65.76,30.61 J8.P$4
USB_VBUS
  Top 0.813: USB2.TOP_VBUS USB2.BOT_VBUS 79.1,91.4 80.01,90.75 83.51,88.5 86.76,88.5 88.51,86.75 FB3.P$2 C26.P$2
  Bottom 0.813: D15.P$2 USB2.TOP_VBUS | USB2.BOT_VBUS D14.P$2
USBB_DM  (via drill 0.38)
  Top 0.254: SAMA1.P$2 68.87,37.26 v68.86,36
  HighSpeed 0.254: v68.86,36 74.76,36 77.01,38.25 77.01,60 79.26,62.25 79.26,82.87 74.02,88.11 USB2.TOP_D_N
  Bottom 0.381: D11.P$2 USB2.TOP_D_N
USBB_DP  (via drill 0.38)
  Top 0.254: SAMA1.P$1 70.37,37.76 v70.36,37
  HighSpeed 0.254: v70.36,37 74.01,37 76.01,39 76.01,60.5 78.26,62.75 78.26,82.27 71.98,88.54 USB2.TOP_D_P
  Bottom 0.381: D10.P$2 USB2.TOP_D_P
USBC_DM  (via drill 0.38)
  Top 0.254: SAMA1.P$4 65.87,37.26 v65.86,35
  HighSpeed 0.254: v65.86,35 75.76,35 78.01,37.25 78.01,59.75 80.26,62 80.26,83.25 75.51,88 77.26,91.25 USB2.BOT_D_N
  Bottom 0.381: D13.P$2 USB2.BOT_D_N
USBC_DP  (via drill 0.38)
  Top 0.254: SAMA1.P$3 67.37,38.36 v67.36,37.85
  HighSpeed 0.254: v67.36,37.85 73.36,37.85 75.01,39.5 75.01,61.25 77.26,63.5 77.26,81.5 70.51,88.25 73.51,93.25 USB2.BOT_D_P
  Bottom 0.381: D12.P$2 USB2.BOT_D_P
V_BACKUP  (via drill 0.38)
  Top 0.203: R1.P$2 25.11,77.35 25.76,78 28.26,78 | 28.26,78 28.86,78 C7.P$2 | U3.P$4 28.22,77.96 28.26,78
  Top 0.254: U3.P$4 v27.26,77 | R3.P$2 | 28.86,78 28.91,78.05 28.91,80.35 28.76,80.5 28.76,80.75 | R2.P$2 25.01,83.25 26.01,84.25 29.51,84.25 | 28.76,80.75 28.76,82.25 28.9,82.4 C8.P$1 | U2.P$8 28.68,80.83 28.76,80.75
  Top 0.381: C8.P$1 29.51,84.25 C58.P$2 36.31,84.06 U14.P$5 | R3.P$2 26.61,73.9 27.61,72.9 27.61,69.45 | 27.61,69.45 27.26,69.1 C9.P$2 33.26,66 | U4.P$6 27.56,69.2 27.61,69.45 | 43.01,56.25 43.01,43.5 44.76,41.75 44.76,40.57 SAMA1.P$18
  Top 0.406: 33.26,66 34.51,66 v38.01,62.5 | v38.01,59 40.26,59 43.01,56.25
  HighSpeed 0.406: v38.01,62.5 v38.01,59
  Bottom 0.254: v27.26,77 27.26,75.15 R3.P$2
  other vias: 26.61,74.5
V_BATT_FUSED
  Top 0.381: C56.P$2 36.31,81.1 | 36.31,81.1 37.95,81.1 38.21,80.85 U14.P$3 U7.P$1 38.8,77.35 C31.P$2 | U14.P$1 36.31,81.1 | 40.76,84.5 40.76,77.25
  Top 0.406: U1.P$2 71.62,80.61 71.86,80.85 C5.P$2 | U10.P$2 51.62,80.61 51.86,80.85 C43.P$2 | 55.01,85.75 42.01,85.75 40.76,84.5 | 40.76,77.25 40.26,76.75 39.61,76.75 C31.P$2
  Top 1.016: 55.01,85.75 C44.P$2 C43.P$2 | 55.01,85.75 72.51,85.75 73.76,84.5 C5.P$2 C6.P$2 78.41,80.85 83.76,75.5 91.41,75.55 99.01,68 99.01,55.5 100.76,53.75 102.99,53.75 J3.P$3 J3.P$4 | 55.01,85.75 PF1.P$2
V_BATT_UNFUSED
  Top 0.406: D16.P$1 39.01,90.88
  Top 0.813: J5.P$1 39.01,90.88 40.13,90.88 40.76,90.25 40.76,88.25 41.51,87.5 47.51,87.5 49.01,89 49.01,95.25 50.51,96.75 PF1.P$1 56.76,96.75 58.01,98 J4.P$1
V_BOOTSTRAP
  Top 0.381: U7.P$5 38.21,73.19 C33.P$2 38.4,70.86 39.26,70 39.26,68.86 D25.AN 39.37,62.89 39.76,62.5 58.26,62.5 59.26,63.5 59.26,67.89 D26.AN
V_MOT
  Top 0.254: 20.01,23.88 U8.P$14 U8.P$13
  Top 0.381: U8.P$24 26.83,25.18 26.01,26 20.26,26 20.01,26.25
  Top 0.813: 20.01,23.88 20.01,26.25 20.01,26.75 18.26,28.5 18.26,41 20.51,43.25 20.51,44.45 C20.P 20.51,44.55 20.51,45.75 21.51,46.75 C19.P$2 C17.P$2 FB1.P$1
V_SHARP  (via drill 0.38)
  Top 0.381: C30.P$2 27.91,43.45 26.65,42.19 26.65,37.64 24.01,35 v21.76,35
  Top 0.406: FB5.P$2 27.26,52.5 27.61,51.65 C29.P$2 27.61,49.29 C30.P$2
  Bottom 0.381: v21.76,35 20.76,35 19.76,34 19.76,30.5 21.76,28.5 32.76,28.5 33.76,27.5 33.76,24.75 34.01,24.5 J1.P$3
VAR_RX  (via drill 0.38)
  Top 0.254: SAMA1.P$53 47.87,11.64 v47.76,11.75
  Shield 0.254: v47.76,11.75 22.76,11.75 20.51,14 18.76,14 13.76,19 13.76,22.25 6.51,29.5 6.51,32.75 5.51,33.75 5.51,46.5 4.26,47.75 2.68,47.75 J2.P$6
VAR_TX  (via drill 0.38)
  Top 0.254: SAMA1.P$54 49.37,11.64 47.76,13.25 v46.76,13.25
  Shield 0.254: v46.76,13.25 22.26,13.25 20.76,14.75 19.01,14.75 14.51,19.25 14.51,22.5 7.26,29.75 7.26,33 6.26,34 6.26,48.75 4.51,50.5 2.55,50.5 J2.P$5
VDD_FUSE
  Top 0.381: U13.P$5 46.7,55.05 C55.P$2 46.37,54.72 SAMA1.P$17

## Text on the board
tPlace: VBAT | GND | Console | 5.0V | 3.3V | SDA | SYS | SCL | PWR | GND | BAT | KEY | BAT | TX | GND | RX | GND | GND | IMU | z | y | x
bPlace: SDA | MAEBot Rev 2.0 APRIL Lab 2013 | SCL | SYS | GND | PWR | KEY | BAT | TX | BAT | RX | GND | GND | GND | GND | NRST | TDO | TCK | TMS | TDI | NTRST | 3.3V | SIG | GND | 5.0V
